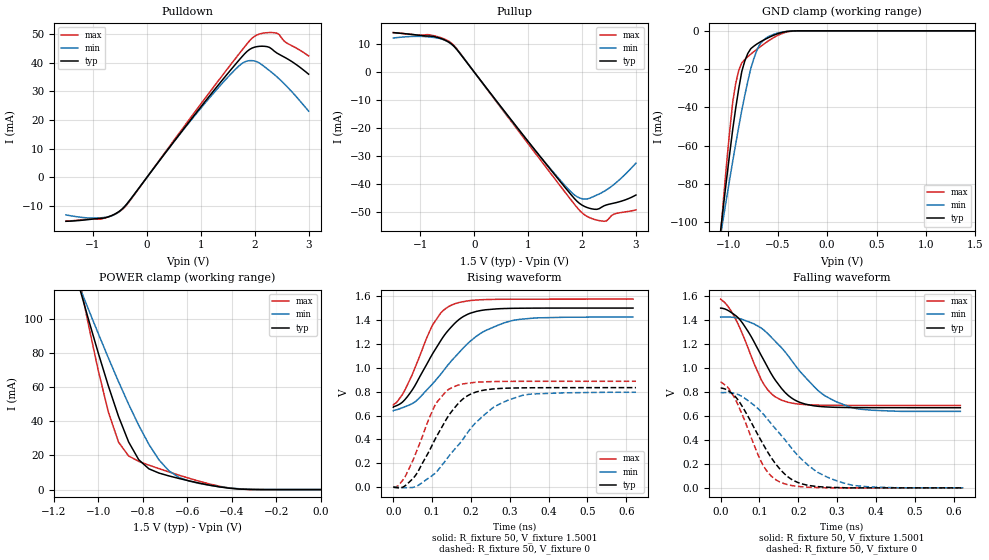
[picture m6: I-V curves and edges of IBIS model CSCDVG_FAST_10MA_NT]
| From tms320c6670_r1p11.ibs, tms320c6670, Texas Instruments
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|   Model Cell CSCDVG_FAST_10MA_NT
|FAST_10MA
[Model]   CSCDVG_FAST_10MA_NT
Model_type   I/O
Polarity   Non-Inverting
Enable   Active-Low
Cref =  4.0000pF
Rref =  100.0000M
Vref =  0V
Vmeas =  0.75
C_comp   1.5249p   1.4275p   1.6205p
|[mode_tieoffpin] SR0=1  SR1=0 I0=0 I1=1 I2=1
[Model Spec]
Vinl   0.6125   0.6125   0.6125
Vinh   0.9625   0.9625   0.9625
D_overshoot_high 1.95 1.95 1.95
D_overshoot_low -0.3 -0.3 -0.3
D_overshoot_time 1E-9 1E-9 1E-9
S_overshoot_high 1.575 1.575 1.575
S_overshoot_low 0 0 0
[Receiver Thresholds]
Reference_supply Pullup_ref
Threshold_sensitivity= 0.5
Tslew_ac= 5nS
Vinh_ac= +175mV
Vinh_dc= +100mV
Vinl_ac= -175mV
Vinl_dc= -100mV
Vth = 0.75
Vth_max= 0.79
Vth_min= 0.71
[Pullup Reference] 1.5001   1.425   1.575
[Add Submodel]
|Submodel_name Mode
CSCDVG_NT Non-Driving
[Temperature Range]   25   105   -40
[Voltage Range]   1.5   1.425   1.575
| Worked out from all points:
|   slope of the pulldown table from 0 to 0.225 V, typ, clamps not added: 39.9 ohm
|   slope of the pullup table from 0 to 0.225 V, typ, clamps not added: 39.8 ohm
|   GND clamp passes 1 mA (typ) near -0.47 V on its own axis
|   POWER clamp passes 1 mA (typ) near -0.42 V on its own axis
|   rising waveform, R_fixture 50, V_fixture 1.5001: 20-80 % time 94.2ps typ, 135ps min, 71.8ps max; typ from 0.669 V to 1.5 V
|   rising waveform, R_fixture 50, V_fixture 0: 20-80 % time 89ps typ, 126ps min, 68ps max; typ from 0 V to 0.834 V
|   falling waveform, R_fixture 50, V_fixture 1.5001: 20-80 % time 90.7ps typ, 130ps min, 71.1ps max; typ from 1.5 V to 0.669 V
|   falling waveform, R_fixture 50, V_fixture 0: 20-80 % time 92.1ps typ, 133ps min, 69.2ps max; typ from 0.833 V to 0 V
[POWER_clamp]
|   voltage   I(typ)   I(min)   I(max)
-1.5V     321.7mA    260.6mA    415.9mA
-1.076V   114.2mA    115.8mA    116.9mA
-1.061V   107.2mA    110.9mA    107.1mA
-954.6mV  60.59mA    77.06mA    45.35mA
-909.2mV  42.85mA    63.21mA    27.81mA
-863.7mV  27.9mA     49.99mA    19.69mA
-818.2mV  17.49mA    37.63mA    16.52mA
-772.8mV  12.19mA    26.53mA    14.33mA
-681.9mV  7.985mA    10.89mA    10.33mA
-590.9mV  5.094mA    4.955mA    6.6mA
-363.7mV  298.5uA    465.2uA    297.6uA
0V        1.518nA    24.08nA    367.8pA
[Pulldown]
|   voltage   I(typ)   I(min)   I(max)
-1.5V     -15.29mA   -13.07mA   -15.28mA
-772.8mV  -14.07mA   -13.9mA    -14.11mA
-590.9mV  -12.74mA   -12.86mA   -12.82mA
-409.1mV  -10.08mA   -10.11mA   -10.32mA
1.046V    25.68mA    25.17mA    26.75mA
1.591V    38.31mA    36.75mA    40.25mA
1.818V    43.24mA    40.36mA    45.69mA
1.955V    45.18mA    40.77mA    48.64mA
2.091V    45.77mA    39.91mA    50.06mA
2.273V    45.4mA     37.32mA    50.56mA
2.364V    44.07mA    35.93mA    50.51mA
3V        36.04mA    23.14mA    42.4mA
[Pullup]
|   voltage   I(typ)   I(min)   I(max)
-1.5V     14.1mA     12.18mA    14.13mA
-818.2mV  12.87mA    12.54mA    13.29mA
-590.9mV  11.83mA    11.72mA    12.11mA
-409.1mV  9.844mA    9.773mA    10.15mA
1.227V    -30.36mA   -30.27mA   -31.43mA
1.727V    -42.29mA   -41.55mA   -44.05mA
1.909V    -46.29mA   -44.65mA   -48.54mA
2.046V    -48.11mA   -45.48mA   -51.1mA
2.227V    -49.12mA   -44.44mA   -52.74mA
2.409V    -47.87mA   -42.71mA   -53.43mA
2.591V    -46.92mA   -40.26mA   -50.87mA
3V        -44.02mA   -32.61mA   -49.35mA
[GND_clamp]
|   voltage   I(typ)   I(min)   I(max)
-1.5V     -310.1mA   -250.5mA   -402.5mA
-1.076V   -103.6mA   -106.2mA   -105.2mA
-1.046V   -89.81mA   -96.36mA   -86.02mA
-954.6mV  -51.22mA   -67.87mA   -36.88mA
-924.3mV  -40.08mA   -58.86mA   -27.29mA
-863.7mV  -21.24mA   -41.56mA   -16.73mA
-833.4mV  -15.8mA    -33.75mA   -15.03mA
-772.8mV  -9.345mA   -19.75mA   -12.19mA
-712.2mV  -6.928mA   -10.35mA   -9.704mA
-621.3mV  -4.261mA   -3.896mA   -6.225mA
-409.1mV  -337.1uA   -289.1uA   -618.9uA
1.5V      1.518nA    257.2nA    299pA
[Ramp]
| variable   typ   min   max
dV/dt_f   0.665384/0.13628682n   0.629864/0.2000188n   0.71/0.10897595n
dV/dt_r  0.6716992/0.13165568n 0.64196624/0.19536277n 0.71221096/0.10400915n
R_load = 50
[Rising Waveform]
R_fixture = 50
V_fixture = 1.5001
V_fixture_min = 1.425
V_fixture_max = 1.575
|   time   V(typ)   V(min)   V(max)
0s        669.3mV    639.1mV    688.4mV
30.11ps   734mV      673.6mV    814.7mV
60.19ps   876.5mV    725.6mV    1.034V
101.7ps   1.12V      866.7mV    1.361V
126.4ps   1.248V     963.5mV    1.473V
155.1ps   1.362V     1.077V     1.532V
191.5ps   1.448V     1.202V     1.561V
225.4ps   1.48V      1.29V      1.57V
302.2ps   1.498V     1.392V     1.574V
617.4ps   1.5V       1.425V     1.575V
[Rising Waveform]
R_fixture = 50
V_fixture = 0
V_fixture_min = 0
V_fixture_max = 0
|   time   V(typ)   V(min)   V(max)
0s        0V         0V         0V
13.22ps   -5.968mV   -2.685mV   12.57mV
27.88ps   5.983mV    -5.338mV   75.12mV
55.63ps   91.65mV    1.606mV    264.6mV
110.1ps   416.3mV    122.5mV    701.4mV
152.1ps   641.7mV    295.4mV    835.8mV
197.7ps   776.9mV    485.3mV    872.8mV
255.3ps   821.9mV    662.3mV    884.2mV
331.6ps   831.8mV    767.8mV    886.4mV
625.1ps   833.5mV    794.6mV    886.9mV
[Falling Waveform]
R_fixture = 50
V_fixture = 1.5001
V_fixture_min = 1.425
V_fixture_max = 1.575
|   time   V(typ)   V(min)   V(max)
0s        1.499V     1.424V     1.575V
26.79ps   1.464V     1.424V     1.477V
52.47ps   1.391V     1.409V     1.311V
112.2ps   1.059V     1.314V     859.2mV
156.4ps   831mV      1.17V      731.9mV
194.4ps   726.9mV    1.012V     701.6mV
250.5ps   680.5mV    813mV      690.3mV
330.6ps   669.9mV    676.5mV    688mV
390.4ps   668.9mV    647.5mV    687.8mV
617.4ps   668.6mV    638.2mV    687.6mV
[Falling Waveform]
R_fixture = 50
V_fixture = 0
V_fixture_min = 0
V_fixture_max = 0
|   time   V(typ)   V(min)   V(max)
0s        832.6mV    794mV      886mV
23.09ps   803.1mV    793.8mV    818.6mV
46.09ps   727.1mV    776.6mV    681.4mV
108.3ps   370.3mV    621mV      194.7mV
151ps     162.9mV    456.7mV    51.46mV
182.2ps   71.61mV    333mV      19.88mV
226.3ps   20.19mV    186.1mV    5.455mV
313ps     2.03mV     44.3mV     0V
387.4ps   0V         6.739mV    0V
625.1ps   0V         0V         0V
